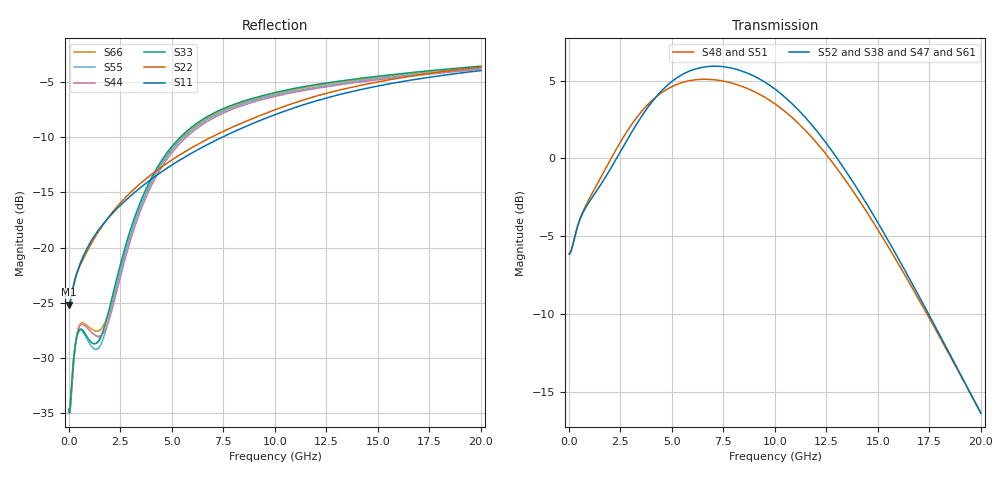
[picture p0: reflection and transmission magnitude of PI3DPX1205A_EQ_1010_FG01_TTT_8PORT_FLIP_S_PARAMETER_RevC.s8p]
! NPort=8 DATA=2000 NOISE=0 GROUPDELAY=0 COMPLEX_DATAFORMAT=POLAR
! NumOfBlock=1 NumOfParam=0
! .MODEL Smodel S TSTONEFILE=PI3DPX1205A_EQ_1010_FG01_TTT_8PORT_FLIP_S_PARAMETER_RevC.s8p TYPE=S
!  -- The above .MODEL line can be used for the S element in the netlist.
! The s parameter is extracted from the linear redriver, it is not bi-directional;
! only s(5,1)s(6,2)s(3,7)s(4,8) should be the insertion loss
!  Port definition:
!  Port1 = AIP
!  Port2 = AIN
!  Port3 = BOP
!  Port4 = BON
!  Port5 = AOP
!  Port6 = AON
!  Port7 = BIP
!  Port8 = BIN
# Hz S MA R  50
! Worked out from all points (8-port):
!   2000 points, 10 MHz to 20 GHz, reference 50 ohm
!   strongest paths, dB at 10 MHz, 5.01 GHz, 10.01 GHz, 15.01 GHz, 20 GHz:
!     S52: -6.1, 5.0, 4.4, -4.2, -16.4
!     S38: -6.1, 4.9, 4.4, -4.2, -16.4
!     S47: -6.1, 4.9, 4.5, -4.1, -16.3
!     S61: -6.1, 4.9, 4.4, -4.1, -16.3
!     S48: -6.1, 4.6, 3.5, -4.6, -16.4
!     S51: -6.1, 4.6, 3.5, -4.6, -16.4
!   lowest |S11| = -25.2 dB at 10 MHz (marker M1), VSWR 1.12, Z = 44.8 - j0.115 ohm
!   |S11| at or under -10 dB: start of sweep to 7.457 GHz
